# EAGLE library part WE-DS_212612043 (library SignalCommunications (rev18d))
WE-DS D-SUB-Filter Connectors Bent 90° Characteristics Standard type filtered with 1000 pF High attenuation of more than 40 dB @ 180 MHz Choice of earthing metal sheet or high speed earthing clip Rated voltage: 100 VDC Rated current @ 20 ºC: 5 A Withstand voltage: 250 VRMS Insulation resistance: min. 1000 MΩ Operating temperature: –55 ºC to +125 ºC Applications Filtering of interfaces External connection to -printer -sensor -display Details see: http://katalog.we-online.de/en/pbs/Filter_abgewinkelt Created on 2015-05-04 2015 (C) Wurth Elektronik
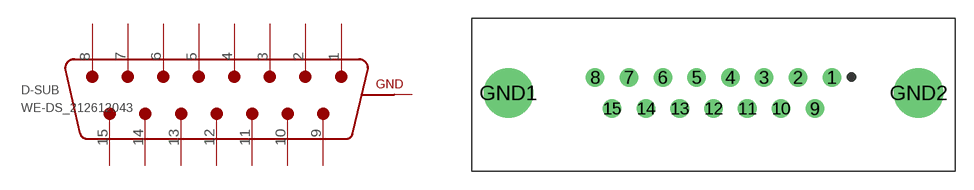
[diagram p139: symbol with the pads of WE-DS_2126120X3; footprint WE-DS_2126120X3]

Designator prefix D-SUB

## WE-DS_212612043 (WE-NUMBER: 212612043/15pins_female)  [WE-DS_2126120X3]
1  8  pas
2  7  pas
3  6  pas
4  5  pas
5  4  pas
6  3  pas
7  2  pas
8  1  pas
9  15  pas
10  14  pas
11  13  pas
12  12  pas
13  11  pas
14  10  pas
15  9  pas
GND1  GND  pas
GND2  GND  pas

## Footprint WE-DS_2126120X3 (pad centres in mm)
drill 1: 1 9.6,1.27; 2 6.86,1.27; 3 4.11,1.27; 4 1.37,1.27; 5 -1.37,1.27; 6 -4.11,1.27; 7 -6.86,1.27; 8 -9.6,1.27; 9 8.23,-1.27; 10 5.48,-1.27; 11 2.74,-1.27; 12 0,-1.27; 13 -2.74,-1.27; 14 -5.48,-1.27; 15 -8.23,-1.27
drill 3: GND1 -16.65,0; GND2 16.65,0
